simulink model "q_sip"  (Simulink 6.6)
settings: Solver=FixedStepDiscrete  StartTime=0.0  StopTime=inf  FixedStep=0.002  RelTol=1e-3
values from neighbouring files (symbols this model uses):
  ALPHA_LIM_ENABLE = 1    [setup_srv02_exp08_sip.m]
  ALPHA_MAX = 45    [setup_srv02_exp08_sip.m]
  ALPHA_MIN = - ALPHA_MAX    (= -45)    [setup_srv02_exp08_sip.m]
  CATCH_ALPHA_DOT_LIM = VMAX_AMP/k(4)    [setup_srv02_exp08_sip.m]
  CATCH_ALPHA_UP_LIM = 1.5 * pi / 180    (= 0.0261799387799)    [setup_srv02_exp08_sip.m]
  eta_g = 0.90    (= 0.9)    [config_srv02.m]
  eta_m = 0.69    [config_srv02.m]
  k = zeros(1,4)    [setup_srv02_exp08_sip.m]
  K_AMP = 1    [setup_srv02_exp08_sip.m]
  K_ENC = 0    [config_srv02.m]
  K_POT = -(352 * pi / 180 / 10)    (= -0.614355896702)    [config_srv02.m]
  K_POT_PEN = -(345 * pi / 180 / 24)    (= -0.250891079974)    [config_sp.m]
  Kg = 0    [config_srv02.m]
  km = 0.804 / 1000 * K_RDPS2RPM    [config_srv02.m]
  kt = 1.088 * K_OZ2N * K_IN2M    [config_srv02.m]
  Rm = 2.6    [config_srv02.m]
  RtpnOff = 0    [config_sp.m]
  RtpnOp = 2    [config_sp.m]
  THETA_LIM_ENABLE = 1    [setup_srv02_exp08_sip.m]
  THETA_MAX = 60    [setup_srv02_exp08_sip.m]
  THETA_MIN = - THETA_MAX    (= -60)    [setup_srv02_exp08_sip.m]
  VMAX_AMP = 0    [config_srv02.m]
  VMAX_DAC = 10    [setup_srv02_exp08_sip.m]
  wcf_1 = 2 * pi * 50.0    (= 314.159265359)    [setup_srv02_exp08_sip.m]
  wcf_2 = 2 * pi * 8.5    (= 53.407075111)    [setup_srv02_exp08_sip.m]
undefined symbols (not defined in the file or in its folder): HIL, qc_get_step_size
libraries: quarc_library x12, simulink_extras x6

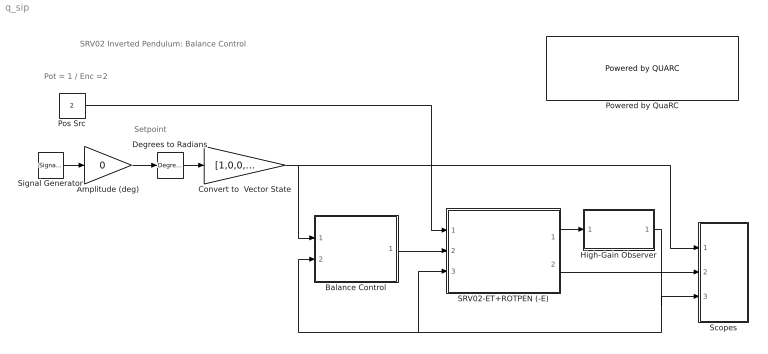
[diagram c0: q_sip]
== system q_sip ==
  note: Setpoint
  note: SRV02 Inverted Pendulum: Balance Control
  note: Pot = 1 / Enc =2
  Amplitude (deg) : Gain  Gain=0
  Balance Control : Subsystem
  Convert to  Vector State : Gain  Gain=[1,0,0,0]
  Degrees to Radians : simulink_extras/Transformations/Degrees to Radians  SystemSampleTime=-1
  High-Gain Observer : Subsystem
  Pos Src : Constant  Value=2
  Powered by QuaRC : quarc_library/Logos/Powered by QUARC  SystemSampleTime=-1
  SRV02-ET+ROTPEN (-E) : Subsystem
  Scopes : Subsystem
  Signal Generator : SignalGenerator  WaveForm=square  Frequency=0.1
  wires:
  Amplitude (deg)/1 -> Degrees to Radians/1
  Signal Generator/1 -> Amplitude (deg)/1
  Degrees to Radians/1 -> Convert to  Vector State/1
  Convert to  Vector State/1 -> Scopes/1(X_d), Balance Control/1(Xd)
  High-Gain Observer/1(Xe) -> Scopes/3(X), Balance Control/2(X), SRV02-ET+ROTPEN (-E)/3(X)
  Balance Control/1(tau (N.m)) -> SRV02-ET+ROTPEN (-E)/2(tau (N.m))
  Pos Src/1 -> SRV02-ET+ROTPEN (-E)/1(srv02 pos src)
  SRV02-ET+ROTPEN (-E)/1(Y) -> High-Gain Observer/1(Y)
  SRV02-ET+ROTPEN (-E)/2(Vm (V)) -> Scopes/2(Vm)

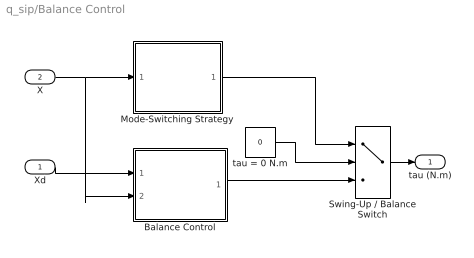
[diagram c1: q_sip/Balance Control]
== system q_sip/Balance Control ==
  Xd : Inport
  X : Inport  Port=2
  Balance Control : Subsystem
  Mode-Switching Strategy : Subsystem
  Swing-Up / Balance Switch : MultiPortSwitch  Inputs=2  zeroidx=on
  tau = 0 N.m : Constant  Value=0
  tau (N.m) : Outport
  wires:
  Swing-Up / Balance Switch/1 -> tau (N.m)/1
  Xd/1 -> Balance Control/1(Xd)
  tau = 0 N.m/1 -> Swing-Up / Balance Switch/2
  X/1 -> Mode-Switching Strategy/1(X), Balance Control/2(X)
  Mode-Switching Strategy/1(enable) -> Swing-Up / Balance Switch/1
  Balance Control/1(tau (N.m)) -> Swing-Up / Balance Switch/3

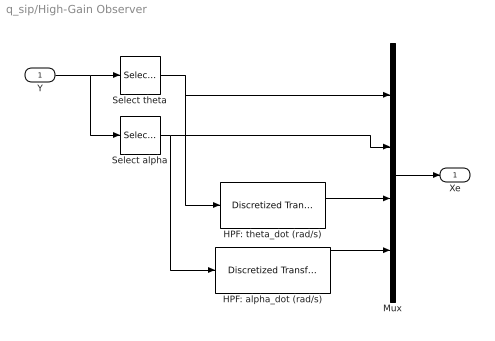
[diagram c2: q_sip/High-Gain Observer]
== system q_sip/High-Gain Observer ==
  Y : Inport
  HPF: alpha_dot (rad/s) : quarc_library/Discrete/Discretized Transfer Function  SystemSampleTime=-1  num=[wcf_2 0]  den=[1 wcf_2]  method=tustin  Ts=qc_get_step_size
  HPF: theta_dot (rad/s) : quarc_library/Discrete/Discretized Transfer Function  SystemSampleTime=-1  num=[wcf_1 0]  den=[1 wcf_1]  method=tustin  Ts=qc_get_step_size
  Mux : Mux
  Select alpha : Selector  IndexOptions=Index vector (dialog)  Indices=2  OutputSizes=[(-2)]  InputPortWidth=2
  Select theta : Selector  IndexOptions=Index vector (dialog)  Indices=1  OutputSizes=[(-2)]  InputPortWidth=2
  Xe : Outport
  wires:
  Select alpha/1 -> Mux/2, HPF: alpha_dot (rad/s)/1
  Mux/1 -> Xe/1
  Y/1 -> Select alpha/1, Select theta/1
  HPF: theta_dot (rad/s)/1 -> Mux/3
  Select theta/1 -> Mux/1, HPF: theta_dot (rad/s)/1
  HPF: alpha_dot (rad/s)/1 -> Mux/4

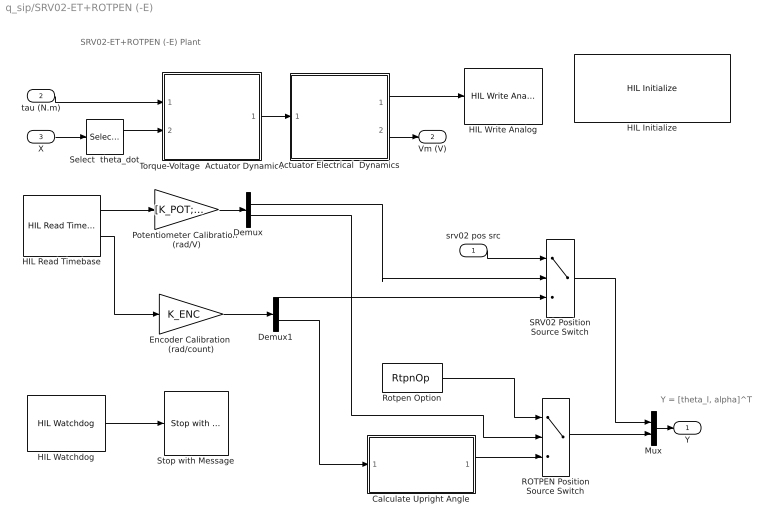
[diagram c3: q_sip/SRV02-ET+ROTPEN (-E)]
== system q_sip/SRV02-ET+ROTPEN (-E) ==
  note: SRV02-ET+ROTPEN (-E) Plant
  note: Y = [theta_l, alpha]^T
  srv02 pos src : Inport
  tau (N.m) : Inport  Port=2
  X : Inport  Port=3
  Actuator Electrical  Dynamics : Subsystem
  Calculate Upright Angle : Subsystem
  Demux : Demux  Outputs=2
  Demux1 : Demux  Outputs=2
  Encoder Calibration  (rad/count) : Gain  Gain=K_ENC
  HIL Initialize : quarc_library/Data Acquisition/Generic/Configuration/HIL Initialize  object_name=HIL-1  board_type=q8  board_number=0  exclusive=off  active=on  hardware_clocks=0:1  clock_modes=[0 0]  set_clock_params_at_start=on  set_clock_params_at_switch_in=off  analog_input_channels=0:7  analog_input_maximums=10  analog_input_minimums=-10  set_analog_input_params_at_start=on  set_analog_input_params_at_switch_in=off  analog_output_channels=0:7  analog_output_maximums=10  analog_output_minimums=-10  initial_analog_outputs=0  final_analog_outputs=0  watchdog_analog_outputs=0  set_analog_output_params_at_start=on  set_analog_output_params_at_switch_in=off  set_analog_outputs_at_start=on  set_analog_outputs_at_switch_in=off  set_analog_outputs_at_terminate=on  set_analog_outputs_at_switch_out=off  set_analog_outputs_on_watchdog=on  digital_input_channels=[]  digital_output_channels=[]  digital_output_configuration=[]  initial_digital_outputs=1  final_digital_outputs=1  watchdog_digital_outputs=0  set_digital_output_params_at_start=off  set_digital_output_params_at_switch_in=off  set_digital_outputs_at_start=on  set_digital_outputs_at_switch_in=off  set_digital_outputs_at_terminate=on  set_digital_outputs_at_switch_out=off  set_digital_outputs_on_watchdog=off  encoder_channels=0:7  quadrature=4  encoder_filter_frequency=(1/120e-9)/1  initial_encoder_counts=0  set_encoder_params_at_start=on  set_encoder_params_at_switch_in=off  set_encoder_counts_at_start=on  set_encoder_counts_at_switch_in=off  pwm_channels=[]  pwm_modes=0  pwm_frequency=(1/60e-9)/1024  pwm_configuration=[]  pwm_alignment=[]  pwm_polarity=[]  pwm_leading_deadband=[]  pwm_trailing_deadband=[]  initial_pwm_outputs=0  final_pwm_outputs=0  watchdog_pwm_outputs=0  set_pwm_params_at_start=on  set_pwm_params_at_switch_in=off  set_pwm_outputs_at_start=on  set_pwm_outputs_at_switch_in=off  set_pwm_outputs_at_terminate=on  set_pwm_outputs_at_switch_out=off  set_pwm_outputs_on_watchdog=off  other_output_channels=[]  initial_other_outputs=[]  final_other_outputs=[]  watchdog_other_outputs=0  set_other_outputs_at_start=on  set_other_outputs_at_switch_in=off  set_other_outputs_at_terminate=on  set_other_outputs_at_switch_out=off  set_other_outputs_on_watchdog=off
  HIL Read Timebase : quarc_library/Data Acquisition/Generic/Timebases/HIL Read Timebase  object_name=HIL-1  clock=0  analog_channels=[0,1]  encoder_channels=[0:1]  digital_channels=[]  other_channels=[]  samples_in_buffer=max(ceil(1/qc_get_step_size), 1)  active=on  vector_output=on  data_type_mode=Inherit via back propagation  encoder_data_type=double  digital_data_type=boolean
  HIL Watchdog : quarc_library/Data Acquisition/Generic/Watchdog/HIL Watchdog  object_name=HIL-1  timeout=10*qc_get_step_size  sample_time=qc_get_step_size  active=off
  HIL Write Analog : quarc_library/Data Acquisition/Generic/Immediate I//O/HIL Write Analog  object_name=HIL-1  channels=0  sample_time=-1  active=off  vector_input=off
  Mux : Mux  Inputs=2
  Potentiometer Calibration  (rad/V) : Gain  Gain="[K_POT;  K_POT_PEN]"
  ROTPEN Position Source Switch : MultiPortSwitch  Inputs=2
  Rotpen Option : Constant  Value=RtpnOp
  SRV02 Position Source Switch : MultiPortSwitch  Inputs=2
  Select  theta_dot : Selector  IndexOptions=Index vector (dialog)  Indices=[3]  OutputSizes=1  InputPortWidth=4
  Stop with Message : quarc_library/Sinks/Error Handling/Stop with Message  SystemSampleTime=-1  message_type=Fixed error message  message_icon=Warning  message=Watchdog expired. Model has been stopped.
  Torque-Voltage  Actuator Dynamics : Subsystem
  Y : Outport  InitialOutput=0
  Vm (V) : Outport  Port=2  InitialOutput=0
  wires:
  Demux/1 -> SRV02 Position Source Switch/2
  Demux1/1 -> SRV02 Position Source Switch/3
  Encoder Calibration  (rad/count)/1 -> Demux1/1
  Potentiometer Calibration  (rad/V)/1 -> Demux/1
  HIL Read Timebase/2 -> Encoder Calibration  (rad/count)/1
  srv02 pos src/1 -> SRV02 Position Source Switch/1
  Actuator Electrical  Dynamics/2(Vm (V)) -> Vm (V)/1
  Actuator Electrical  Dynamics/1(Vdaq (V)) -> HIL Write Analog/1
  HIL Read Timebase/1 -> Potentiometer Calibration  (rad/V)/1
  SRV02 Position Source Switch/1 -> Mux/1
  Mux/1 -> Y/1
  Demux/2 -> ROTPEN Position Source Switch/2
  Demux1/2 -> Calculate Upright Angle/1(alpha (rad))
  Calculate Upright Angle/1(alpha_up (rad)) -> ROTPEN Position Source Switch/3
  Rotpen Option/1 -> ROTPEN Position Source Switch/1
  ROTPEN Position Source Switch/1 -> Mux/2
  tau (N.m)/1 -> Torque-Voltage  Actuator Dynamics/1(tau (N.m))
  X/1 -> Select  theta_dot/1
  Torque-Voltage  Actuator Dynamics/1(Vi (V)) -> Actuator Electrical  Dynamics/1(Vi (V))
  Select  theta_dot/1 -> Torque-Voltage  Actuator Dynamics/2(th_dot (rad/s))
  HIL Watchdog/1 -> Stop with Message/1

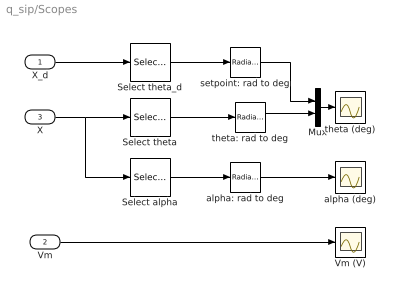
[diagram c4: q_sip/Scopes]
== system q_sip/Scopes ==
  X_d : Inport
  Vm : Inport  Port=2
  X : Inport  Port=3
  Mux : Mux  Inputs=2
  Select alpha : Selector  IndexOptions=Index vector (dialog)  Indices=2  OutputSizes=[(-2)]  InputPortWidth=4
  Select theta : Selector  IndexOptions=Index vector (dialog)  Indices=1  OutputSizes=[(-2)]  InputPortWidth=4
  Select theta_d : Selector  IndexOptions=Index vector (dialog)  Indices=1  OutputSizes=[(-2)]  InputPortWidth=4
  Vm (V) : Scope
  alpha (deg) : Scope
  alpha: rad to deg : simulink_extras/Transformations/Radians to Degrees  SystemSampleTime=-1
  setpoint: rad to deg : simulink_extras/Transformations/Radians to Degrees  SystemSampleTime=-1
  theta (deg) : Scope
  theta: rad to deg : simulink_extras/Transformations/Radians to Degrees  SystemSampleTime=-1
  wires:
  Vm/1 -> Vm (V)/1
  X_d/1 -> Select theta_d/1
  Mux/1 -> theta (deg)/1
  theta: rad to deg/1 -> Mux/2
  Select alpha/1 -> alpha: rad to deg/1
  Select theta/1 -> theta: rad to deg/1
  alpha: rad to deg/1 -> alpha (deg)/1
  X/1 -> Select alpha/1, Select theta/1
  setpoint: rad to deg/1 -> Mux/1
  Select theta_d/1 -> setpoint: rad to deg/1

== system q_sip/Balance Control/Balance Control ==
  Xd : Inport
  X : Inport  Port=2
  PD  Control Gain : Gain  Gain=k  Multiplication=Matrix(K*u)
  Sum : Sum  Inputs=+-
  tau (N.m) : Outport
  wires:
  Sum/1 -> PD  Control Gain/1
  X/1 -> Sum/2
  Xd/1 -> Sum/1
  PD  Control Gain/1 -> tau (N.m)/1

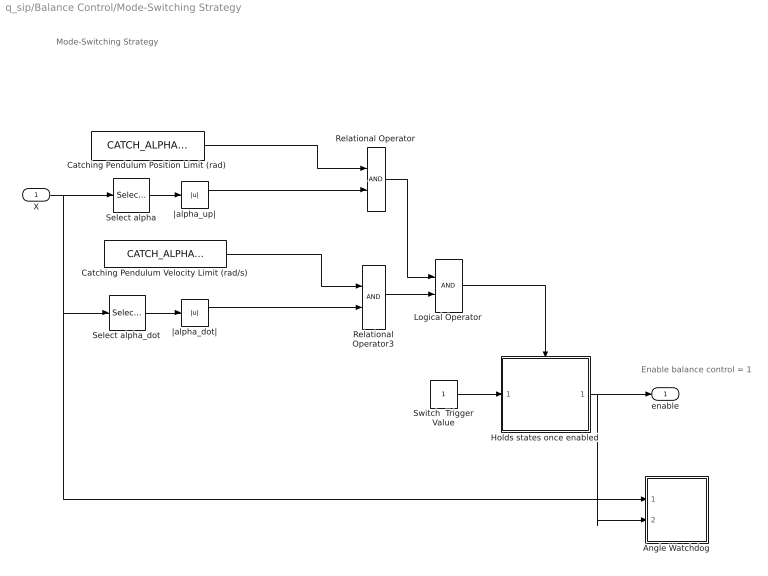
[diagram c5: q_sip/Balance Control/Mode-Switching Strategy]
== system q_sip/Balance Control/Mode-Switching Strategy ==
  note: Mode-Switching Strategy
  note: Enable balance control = 1
  X : Inport
  Angle Watchdog : Subsystem
  Catching Pendulum Position Limit (rad) : Constant  Value=CATCH_ALPHA_UP_LIM
  Catching Pendulum Velocity Limit (rad/s) : Constant  Value=CATCH_ALPHA_DOT_LIM
  Holds states once enabled : Subsystem  TreatAsAtomicUnit=on
  Logical Operator : Logic
  Relational Operator : RelationalOperator
  Relational Operator3 : RelationalOperator
  Select alpha : Selector  IndexOptions=Index vector (dialog)  Indices=2  OutputSizes=[(-2)]  InputPortWidth=4
  Select alpha_dot : Selector  IndexOptions=Index vector (dialog)  Indices=4  OutputSizes=[(-2)]  InputPortWidth=4
  Switch  Trigger Value : Constant
  |alpha_dot| : Abs
  |alpha_up| : Abs
  enable : Outport
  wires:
  Catching Pendulum Position Limit (rad)/1 -> Relational Operator/1
  Logical Operator/1 -> Holds states once enabled/Enable
  Relational Operator/1 -> Logical Operator/1
  Relational Operator3/1 -> Logical Operator/2
  Select alpha_dot/1 -> |alpha_dot|/1
  Catching Pendulum Velocity Limit (rad/s)/1 -> Relational Operator3/1
  |alpha_dot|/1 -> Relational Operator3/2
  Holds states once enabled/1(Sw Trigger) -> enable/1, Angle Watchdog/2(enable)
  Switch  Trigger Value/1 -> Holds states once enabled/1(Trigger)
  Select alpha/1 -> |alpha_up|/1
  |alpha_up|/1 -> Relational Operator/2
  X/1 -> Select alpha/1, Select alpha_dot/1, Angle Watchdog/1(X)

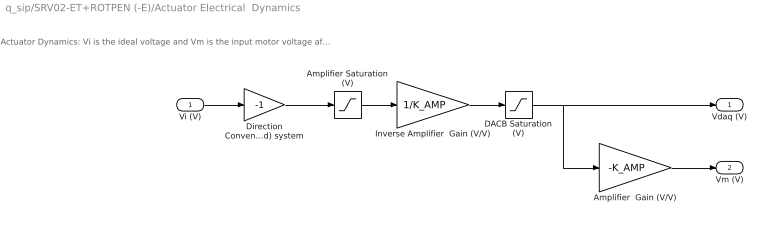
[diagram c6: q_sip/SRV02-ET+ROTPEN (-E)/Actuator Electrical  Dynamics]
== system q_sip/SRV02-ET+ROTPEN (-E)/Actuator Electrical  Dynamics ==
  note: Actuator Dynamics: Vi is the ideal voltage and Vm is the input motor voltage after going through the DACB and amplifier limitiations.
  Vi (V) : Inport
  Amplifier Saturation (V) : Saturate  UpperLimit=VMAX_AMP  LowerLimit=-VMAX_AMP
  Amplifier  Gain (V/V) : Gain  Gain=-K_AMP
  DACB Saturation (V) : Saturate  UpperLimit=VMAX_DAC  LowerLimit=-VMAX_DAC
  Direction Convention: (Right-Hand) system : Gain  Gain=-1
  Inverse Amplifier  Gain (V/V) : Gain  Gain=1/K_AMP
  Vdaq (V) : Outport
  Vm (V) : Outport  Port=2
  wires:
  Direction Convention: (Right-Hand) system/1 -> Amplifier Saturation (V)/1
  Amplifier  Gain (V/V)/1 -> Vm (V)/1
  DACB Saturation (V)/1 -> Vdaq (V)/1, Amplifier  Gain (V/V)/1
  Inverse Amplifier  Gain (V/V)/1 -> DACB Saturation (V)/1
  Amplifier Saturation (V)/1 -> Inverse Amplifier  Gain (V/V)/1
  Vi (V)/1 -> Direction Convention: (Right-Hand) system/1

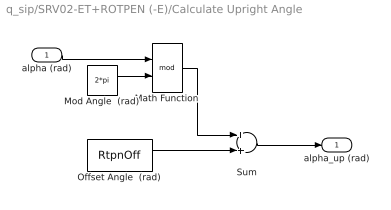
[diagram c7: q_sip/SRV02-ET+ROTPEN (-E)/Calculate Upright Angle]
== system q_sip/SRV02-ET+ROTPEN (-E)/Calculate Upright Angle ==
  alpha (rad) : Inport
  Math Function : Math  Operator=mod
  Mod Angle  (rad) : Constant  Value=2*pi
  Offset Angle  (rad) : Constant  Value=RtpnOff
  Sum : Sum
  alpha_up (rad) : Outport
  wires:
  Sum/1 -> alpha_up (rad)/1
  Mod Angle  (rad)/1 -> Math Function/2
  Offset Angle  (rad)/1 -> Sum/2
  alpha (rad)/1 -> Math Function/1
  Math Function/1 -> Sum/1

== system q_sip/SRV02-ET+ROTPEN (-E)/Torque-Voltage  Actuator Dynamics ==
  tau (N.m) : Inport
  th_dot (rad/s) : Inport  Port=2
  Back-EMF (V.s/rad) : Gain  Gain=Kg*km
  Torque to Voltage (V/(N.m)) : Gain  Gain=Rm / ( eta_g * Kg * eta_m * kt )
  Vi : Sum  OutScaling=2^-10
  Vi (V) : Outport
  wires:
  Vi/1 -> Vi (V)/1
  Back-EMF (V.s/rad)/1 -> Vi/2
  Torque to Voltage (V/(N.m))/1 -> Vi/1
  th_dot (rad/s)/1 -> Back-EMF (V.s/rad)/1
  tau (N.m)/1 -> Torque to Voltage (V/(N.m))/1

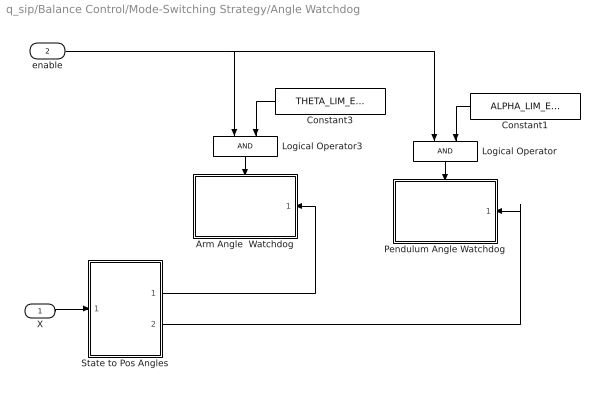
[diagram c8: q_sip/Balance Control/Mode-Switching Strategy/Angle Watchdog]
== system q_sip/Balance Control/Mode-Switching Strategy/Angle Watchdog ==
  X : Inport
  enable : Inport  Port=2
  Arm Angle  Watchdog : Subsystem  Orientation=left  TreatAsAtomicUnit=on
  Constant1 : Constant  Orientation=left  Value=ALPHA_LIM_ENABLE
  Constant3 : Constant  Orientation=left  Value=THETA_LIM_ENABLE
  Logical Operator : Logic  Orientation=down
  Logical Operator3 : Logic  Orientation=down
  Pendulum Angle Watchdog : Subsystem  Orientation=left  TreatAsAtomicUnit=on
  State to Pos Angles : Subsystem
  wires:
  State to Pos Angles/2(alpha (rad)) -> Pendulum Angle Watchdog/1(alpha (rad))
  State to Pos Angles/1(theta (rad)) -> Arm Angle  Watchdog/1(theta (rad))
  enable/1 -> Logical Operator/1, Logical Operator3/1
  X/1 -> State to Pos Angles/1(X)
  Logical Operator/1 -> Pendulum Angle Watchdog/Enable
  Constant1/1 -> Logical Operator/2
  Logical Operator3/1 -> Arm Angle  Watchdog/Enable
  Constant3/1 -> Logical Operator3/2

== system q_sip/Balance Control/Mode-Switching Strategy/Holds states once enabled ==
  Trigger : Inport
  Enable : EnablePort
  Sw Trigger : Outport  InitialOutput=[0]
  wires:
  Trigger/1 -> Sw Trigger/1

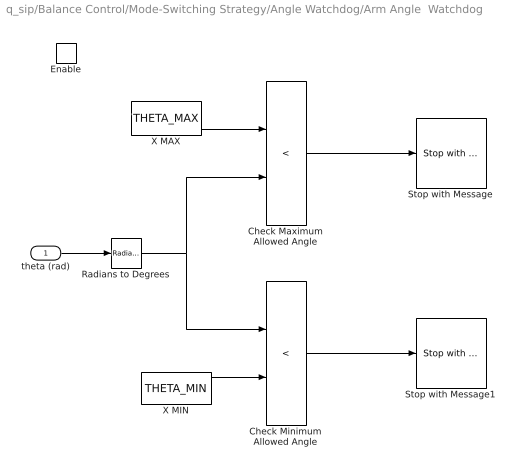
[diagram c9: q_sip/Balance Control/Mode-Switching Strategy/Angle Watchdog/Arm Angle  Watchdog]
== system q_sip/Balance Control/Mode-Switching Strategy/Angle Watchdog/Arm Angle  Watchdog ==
  theta (rad) : Inport
  Enable : EnablePort
  Check Maximum Allowed Angle : RelationalOperator  Operator=<
  Check Minimum Allowed Angle : RelationalOperator  Operator=<
  Radians to Degrees : simulink_extras/Transformations/Radians to Degrees  SystemSampleTime=-1
  Stop with Message : quarc_library/Sinks/Error Handling/Stop with Message  SystemSampleTime=-1  message_type=Fixed error message  message_icon=Error  message=Maximum arm angle reached.
  Stop with Message1 : quarc_library/Sinks/Error Handling/Stop with Message  SystemSampleTime=-1  message_type=Fixed error message  message_icon=Error  message=Minimum arm angle reached.
  X MAX : Constant  Value=THETA_MAX
  X MIN : Constant  Value=THETA_MIN
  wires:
  Radians to Degrees/1 -> Check Minimum Allowed Angle/1, Check Maximum Allowed Angle/2
  Check Maximum Allowed Angle/1 -> Stop with Message/1
  theta (rad)/1 -> Radians to Degrees/1
  X MIN/1 -> Check Minimum Allowed Angle/2
  Check Minimum Allowed Angle/1 -> Stop with Message1/1
  X MAX/1 -> Check Maximum Allowed Angle/1

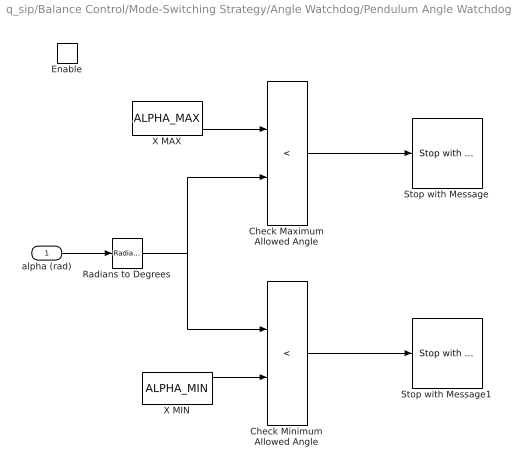
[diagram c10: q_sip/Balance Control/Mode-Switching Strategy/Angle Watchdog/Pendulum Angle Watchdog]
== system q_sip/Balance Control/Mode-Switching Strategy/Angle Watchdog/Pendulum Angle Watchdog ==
  alpha (rad) : Inport
  Enable : EnablePort
  Check Maximum Allowed Angle : RelationalOperator  Operator=<
  Check Minimum Allowed Angle : RelationalOperator  Operator=<
  Radians to Degrees : simulink_extras/Transformations/Radians to Degrees  SystemSampleTime=-1
  Stop with Message : quarc_library/Sinks/Error Handling/Stop with Message  SystemSampleTime=-1  message_type=Fixed error message  message_icon=Error  message=Maximum pendulum angle reached.
  Stop with Message1 : quarc_library/Sinks/Error Handling/Stop with Message  SystemSampleTime=-1  message_type=Fixed error message  message_icon=Error  message=Minimum pendulum angle reached.
  X MAX : Constant  Value=ALPHA_MAX
  X MIN : Constant  Value=ALPHA_MIN
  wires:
  X MAX/1 -> Check Maximum Allowed Angle/1
  Check Minimum Allowed Angle/1 -> Stop with Message1/1
  X MIN/1 -> Check Minimum Allowed Angle/2
  alpha (rad)/1 -> Radians to Degrees/1
  Check Maximum Allowed Angle/1 -> Stop with Message/1
  Radians to Degrees/1 -> Check Maximum Allowed Angle/2, Check Minimum Allowed Angle/1

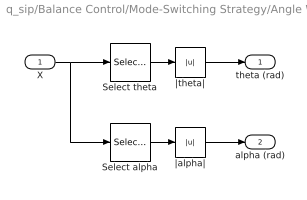
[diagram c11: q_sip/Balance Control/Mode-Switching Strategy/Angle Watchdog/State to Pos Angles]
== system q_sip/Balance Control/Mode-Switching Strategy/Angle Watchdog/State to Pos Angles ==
  X : Inport
  Select alpha : Selector  IndexOptions=Index vector (dialog)  Indices=2  OutputSizes=[(-2)]  InputPortWidth=4
  Select theta : Selector  IndexOptions=Index vector (dialog)  Indices=1  OutputSizes=[(-2)]  InputPortWidth=4
  |alpha| : Abs
  |theta| : Abs
  theta (rad) : Outport
  alpha (rad) : Outport  Port=2
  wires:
  Select alpha/1 -> |alpha|/1
  Select theta/1 -> |theta|/1
  X/1 -> Select alpha/1, Select theta/1
  |theta|/1 -> theta (rad)/1
  |alpha|/1 -> alpha (rad)/1
